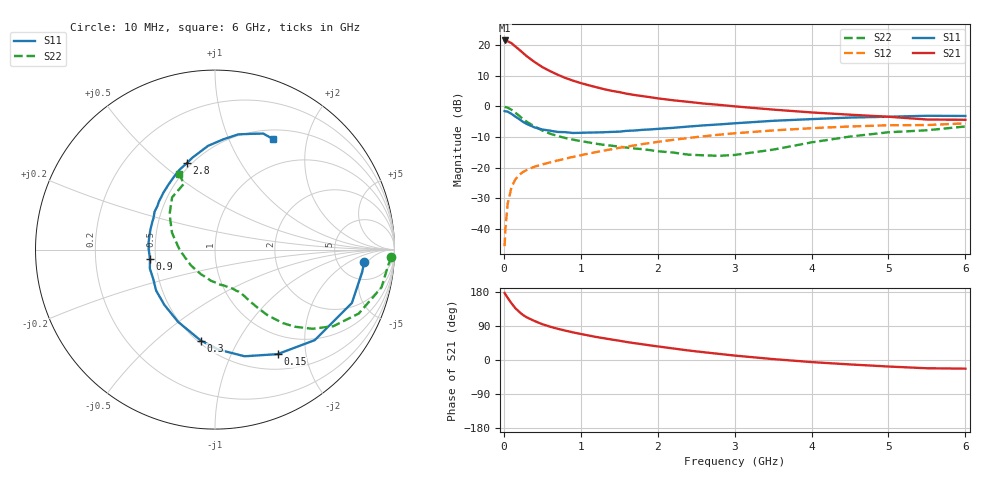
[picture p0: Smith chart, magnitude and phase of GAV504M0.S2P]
! Infineon Technologies  Discrete & RF Semiconductors
! BF775
! Si NPN RF Bipolar Junction Transistor in SOT23
! VCE = 0.5 V  IC = 4 mA
! Common Emitter S-Parameters:  May  1996
# GHz  S  MA  R  50
!  f  S11  S21  S12  S22
! GHz  MAG  ANG  MAG  ANG  MAG  ANG  MAG  ANG
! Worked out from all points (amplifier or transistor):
!   36 points, 10 MHz to 6 GHz, reference 50 ohm
!   highest |S21| = 21.5 dB at 10 MHz (marker M1)
!   |S21| within 3 dB of that: start of sweep to 200 MHz
!   unconditionally stable (mu >= 1): 717.5 MHz to end of sweep
!   at 250 MHz: K = 0.47, MSG = 19.4 dB, |S12| = -21.4 dB
!   at 1.4 GHz: K = 1.23, MAG = 6.6 dB, |S12| = -14.0 dB
!   at 6 GHz: K = 1.09, MAG = -1.2 dB, |S12| = -5.6 dB
!   S11 on the Smith chart (normalised r, x): 10 MHz: 9, -4; 150 MHz: 0.71, -1.53; 300 MHz: 0.52, -0.71; 900 MHz: 0.47, -0.06; 2.8 GHz: 0.47, +0.61; 6 GHz: 0.61, +1.47
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0.01  0.8343 -4.6  11.88 177.0  0.0052 85.9  0.9828 -2.5
0.02  0.8295 -8.7  11.76 173.4  0.0101 86.0  0.969 -5.2
0.05  0.8187 -21.3  11.5 164.0  0.0258 78.4  0.9512 -12.8
0.1  0.7506 -42.2  10.73 149.5  0.0479 67.9  0.8765 -24.0
0.15  0.6788 -59.1  9.462 136.7  0.064 59.9  0.7853 -32.9
0.2  0.6167 -74.5  8.414 127.0  0.0759 54.6  0.6995 -39.1
0.25  0.5575 -88.0  7.413 118.6  0.0847 50.5  0.6186 -44.0
0.3  0.5128 -98.9  6.537 112.4  0.0916 48.4  0.5568 -47.3
0.4  0.452 -117.1  5.282 102.8  0.1033 45.7  0.4689 -51.3
0.5  0.4177 -132.5  4.373 94.5  0.1124 45.0  0.4028 -53.7
0.6  0.3998 -145.1  3.755 88.0  0.1214 44.8  0.3573 -55.5
0.7  0.381 -154.6  3.282 82.4  0.1305 45.2  0.327 -56.8
0.9  0.3663 -171.5  2.619 72.9  0.1492 45.4  0.2856 -59.1
1.1  0.372 173.9  2.211 64.8  0.1687 45.8  0.2574 -62.7
1.3  0.377 162.2  1.908 57.4  0.1891 45.7  0.235 -66.5
1.6  0.3975 147.9  1.603 47.4  0.2199 44.4  0.2112 -74.1
2.2  0.4449 125.7  1.254 30.5  0.283 39.8  0.1758 -96.8
2.8  0.5061 108.1  1.056 16.1  0.344 33.2  0.1553 -133.7
3.5  0.5795 93.8  0.883 2.4  0.4035 24.0  0.1959 -178.8
4.5  0.6549 78.6  0.729 -11.7  0.4682 11.1  0.3206 142.1
5.5  0.7003 67.4  0.608 -21.8  0.4937 -1.9  0.4059 115.2
6  0.6955 62.5  0.602 -22.8  0.5269 -5.4  0.4686 115.5
